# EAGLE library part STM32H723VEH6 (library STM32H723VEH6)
High-performance and DSP with DP-FPU, Arm Cortex-M7 MCU with 512 Kbytes Flash, 564 Kbytes RAM, 550 MHz CPU, L1 cache, external memory interface, subset of peripherals Source: Datasheet
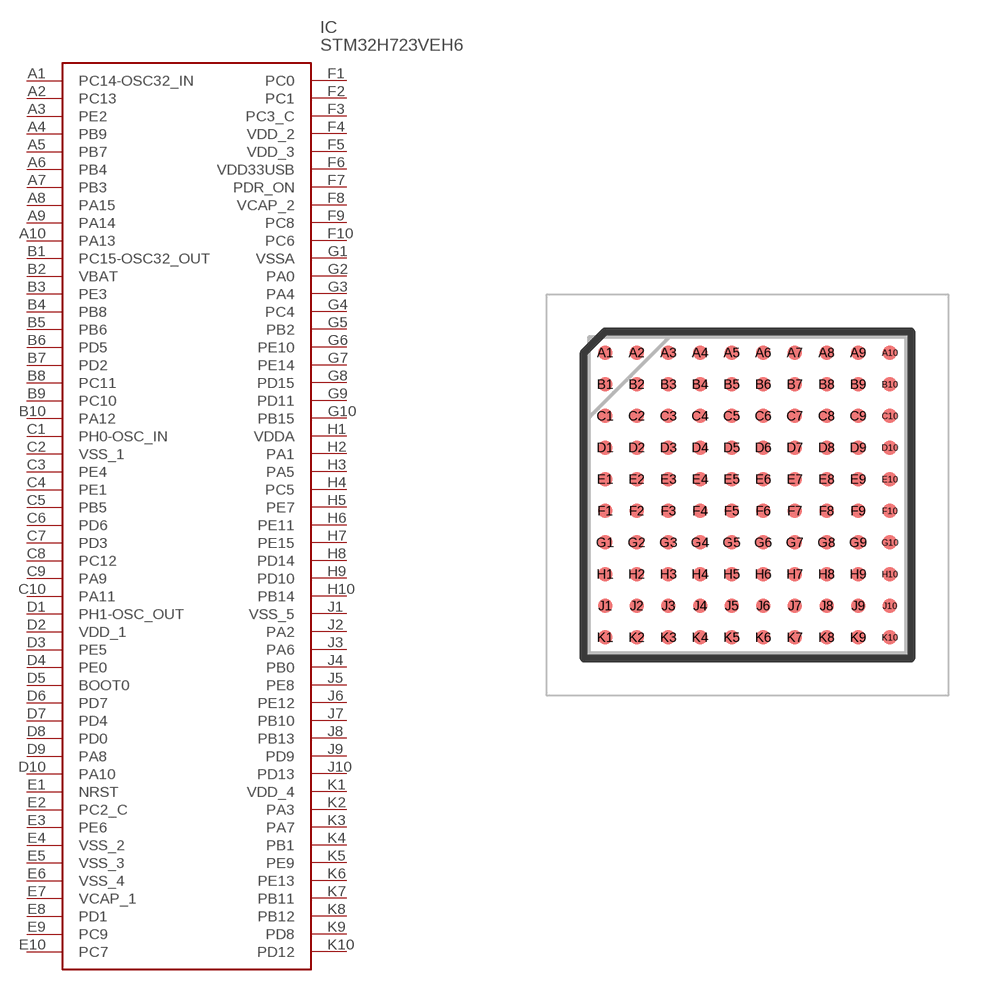
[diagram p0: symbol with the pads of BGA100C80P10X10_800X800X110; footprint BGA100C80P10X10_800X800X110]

Designator prefix IC

## STM32H723VEH6 (Arrow_Part_Number: STM32H723VEH6; Arrow_Price-Stock: https://www.arrow.com/en/products/stm32h723veh6/stmicroelectronics?utm_currency=USD&region=nac; Description: High-performance and DSP with DP-FPU, Arm Cortex-M7 MCU with 512 Kbytes Flash, 564 Kbytes RAM, 550 MHz CPU, L1 cache, external memory interface, subset of peripherals; Height: 1.1mm; Manufacturer_Name: STMicroelectronics; Manufacturer_Part_Number: STM32H723VEH6; Mouser_Part_Number: 511-STM32H723VEH6; Mouser_Price-Stock: https://www.mouser.co.uk/ProductDetail/STMicroelectronics/STM32H723VEH6?qs=sPbYRqrBIVmfnFltjZixRA%3D%3D)  [BGA100C80P10X10_800X800X110]
A1  PC14-OSC32_IN
A2  PC13
A3  PE2
A4  PB9
A5  PB7
A6  PB4
A7  PB3
A8  PA15
A9  PA14
A10  PA13
B1  PC15-OSC32_OUT
B2  VBAT
B3  PE3
B4  PB8
B5  PB6
B6  PD5
B7  PD2
B8  PC11
B9  PC10
B10  PA12
C1  PH0-OSC_IN
C2  VSS_1
C3  PE4
C4  PE1
C5  PB5
C6  PD6
C7  PD3
C8  PC12
C9  PA9
C10  PA11
D1  PH1-OSC_OUT
D2  VDD_1
D3  PE5
D4  PE0
D5  BOOT0
D6  PD7
D7  PD4
D8  PD0
D9  PA8
D10  PA10
E1  NRST
E2  PC2_C
E3  PE6
E4  VSS_2
E5  VSS_3
E6  VSS_4
E7  VCAP_1
E8  PD1
E9  PC9
E10  PC7
F1  PC0
F2  PC1
F3  PC3_C
F4  VDD_2
F5  VDD_3
F6  VDD33USB
F7  PDR_ON
F8  VCAP_2
F9  PC8
F10  PC6
G1  VSSA
G2  PA0
G3  PA4
G4  PC4
G5  PB2
G6  PE10
G7  PE14
G8  PD15
G9  PD11
G10  PB15
H1  VDDA
H2  PA1
H3  PA5
H4  PC5
H5  PE7
H6  PE11
H7  PE15
H8  PD14
H9  PD10
H10  PB14
J1  VSS_5
J2  PA2
J3  PA6
J4  PB0
J5  PE8
J6  PE12
J7  PB10
J8  PB13
J9  PD9
J10  PD13
K1  VDD_4
K2  PA3
K3  PA7
K4  PB1
K5  PE9
K6  PE13
K7  PB11
K8  PB12
K9  PD8
K10  PD12

## Footprint BGA100C80P10X10_800X800X110 (pad centres in mm)
TFBGA 100 8x8x1.2 P 0.8 mm_2022
smd 0.37 x 0.37: A1 -3.6,3.6; A2 -2.8,3.6; A3 -2,3.6; A4 -1.2,3.6; A5 -0.4,3.6; A6 0.4,3.6; A7 1.2,3.6; A8 2,3.6; A9 2.8,3.6; A10 3.6,3.6; B1 -3.6,2.8; B2 -2.8,2.8; B3 -2,2.8; B4 -1.2,2.8; B5 -0.4,2.8; B6 0.4,2.8; B7 1.2,2.8; B8 2,2.8; B9 2.8,2.8; B10 3.6,2.8; C1 -3.6,2; C2 -2.8,2; C3 -2,2; C4 -1.2,2; C5 -0.4,2; C6 0.4,2; C7 1.2,2; C8 2,2; C9 2.8,2; C10 3.6,2; D1 -3.6,1.2; D2 -2.8,1.2; D3 -2,1.2; D4 -1.2,1.2; D5 -0.4,1.2; D6 0.4,1.2; D7 1.2,1.2; D8 2,1.2; D9 2.8,1.2; D10 3.6,1.2; E1 -3.6,0.4; E2 -2.8,0.4; E3 -2,0.4; E4 -1.2,0.4; E5 -0.4,0.4; E6 0.4,0.4; E7 1.2,0.4; E8 2,0.4; E9 2.8,0.4; E10 3.6,0.4; F1 -3.6,-0.4; F2 -2.8,-0.4; F3 -2,-0.4; F4 -1.2,-0.4; F5 -0.4,-0.4; F6 0.4,-0.4; F7 1.2,-0.4; F8 2,-0.4; F9 2.8,-0.4; F10 3.6,-0.4; G1 -3.6,-1.2; G2 -2.8,-1.2; G3 -2,-1.2; G4 -1.2,-1.2; G5 -0.4,-1.2; G6 0.4,-1.2; G7 1.2,-1.2; G8 2,-1.2; G9 2.8,-1.2; G10 3.6,-1.2; H1 -3.6,-2; H2 -2.8,-2; H3 -2,-2; H4 -1.2,-2; H5 -0.4,-2; H6 0.4,-2; H7 1.2,-2; H8 2,-2; H9 2.8,-2; H10 3.6,-2; J1 -3.6,-2.8; J2 -2.8,-2.8; J3 -2,-2.8; J4 -1.2,-2.8; J5 -0.4,-2.8; J6 0.4,-2.8; J7 1.2,-2.8; J8 2,-2.8; J9 2.8,-2.8; J10 3.6,-2.8; K1 -3.6,-3.6; K2 -2.8,-3.6; K3 -2,-3.6; K4 -1.2,-3.6; K5 -0.4,-3.6; K6 0.4,-3.6; K7 1.2,-3.6; K8 2,-3.6; K9 2.8,-3.6; K10 3.6,-3.6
